TYPE ProcessRecipeFeedBack :
STRUCT
	//start process
	ProcessStart :BOOL;
	//finish process
	ProcessFinished :BOOL;
	//process error code
	ProcessError :INT;//0:	1:	2:
	//current step No
	CurrentStepNo :INT;
	CurrentStepstart :BOOL;
	CurrentStepFinished :BOOL;
END_STRUCT
END_TYPE
